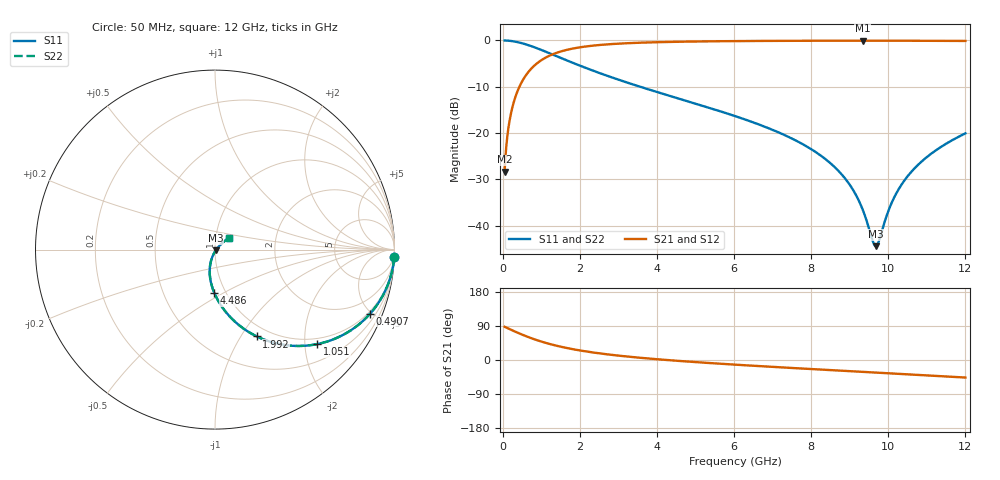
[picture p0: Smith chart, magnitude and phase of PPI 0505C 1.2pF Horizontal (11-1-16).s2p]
# MHz S MA R 50
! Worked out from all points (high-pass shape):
!   1601 points, 50 MHz to 12 GHz, reference 50 ohm
!   highest |S21| = -0.06 dB at 9.334 GHz (marker M1); lowest = -28.3 dB at 50 MHz (marker M2)
!   |S21| within 3 dB of the highest: 1.279 GHz to end of sweep
!   lowest |S11| = -44.4 dB at 9.677 GHz (marker M3), VSWR 1.01, Z = 50.5 - j0.341 ohm
!   |S11| at or under -10 dB: 3.565 GHz to end of sweep
!   |S22| runs from -44.4 to 0.0 dB; largest |S21 - S12| = 0
!   S11 on the Smith chart (normalised r, x): 50 MHz: 1, -48; 490.7 MHz: 0.86, -4.90; 1.051 GHz: 0.86, -2.28; 1.992 GHz: 0.87, -1.17; 4.486 GHz: 0.88, -0.45; 12 GHz: 1.16, +0.15
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50  0.9993 -2.4  0.03837 87.6  0.03837 87.6  0.9993 -2.4
147.0938  0.9937 -7.0  0.1123 83.0  0.1123 83.0  0.9937 -7.0
221.7812  0.9857 -10.5  0.1679 79.5  0.1679 79.5  0.9857 -10.5
341.2812  0.9672 -15.9  0.2537 74.1  0.2537 74.1  0.9672 -15.9
490.6562  0.9354 -22.4  0.353 67.6  0.353 67.6  0.9354 -22.4
1050.812  0.7754 -42.8  0.6299 47.1  0.6299 47.1  0.7754 -42.8
1991.875  0.5365 -64.3  0.8414 25.4  0.8414 25.4  0.5365 -64.3
2044.156  0.5261 -65.2  0.8479 24.5  0.8479 24.5  0.5261 -65.2
2895.594  0.3904 -76.8  0.9175 12.8  0.9175 12.8  0.3904 -76.8
4038.312  0.2746 -87.5  0.9578 1.7  0.9578 1.7  0.2746 -87.5
4486.438  0.2411 -90.9  0.9665 -1.8  0.9665 -1.8  0.2411 -90.9
6025  0.1526 -100.6  0.9836 -12.3  0.9836 -12.3  0.1526 -100.6
8019.156  0.0663 -109.5  0.9921 -24.0  0.9921 -24.0  0.0663 -109.5
8825.781  0.03446 -109.2  0.9933 -28.5  0.9933 -28.5  0.03446 -109.2
9333.656  0.01502 -98.4  0.9935 -31.3  0.9935 -31.3  0.01502 -98.4
9595.062  0.006869 -62.4  0.9934 -32.8  0.9934 -32.8  0.006869 -62.4
9677.219  0.006013 -34.2  0.9934 -33.2  0.9934 -33.2  0.006013 -34.2
9759.375  0.006851 -5.8  0.9933 -33.7  0.9933 -33.7  0.006851 -5.8
10013.31  0.01484 30.3  0.9931 -35.1  0.9931 -35.1  0.01484 30.3
10319.53  0.02679 39.5  0.9927 -36.8  0.9927 -36.8  0.02679 39.5
10737.78  0.04397 42.3  0.9918 -39.1  0.9918 -39.1  0.04397 42.3
12000  0.09923 39.5  0.9871 -46.3  0.9871 -46.3  0.09923 39.5
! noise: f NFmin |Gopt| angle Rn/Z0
50  0.001054  0.9646  1.622  0.006731
1372  0.005839  0.7687  6.755  0.005124
2701  0.00921  0.7178  11.01  0.006397
4031  0.01219  0.6882  15.35  0.007467
5360  0.01499  0.6688  19.68  0.008453
6682  0.01771  0.656  23.92  0.009412
8012  0.02044  0.6481  28.11  0.0104
9341  0.02321  0.644  32.21  0.01144
1.067e+04  0.02608  0.6433  36.19  0.01256
1.2e+04  0.02909  0.6455  40.07  0.01381
